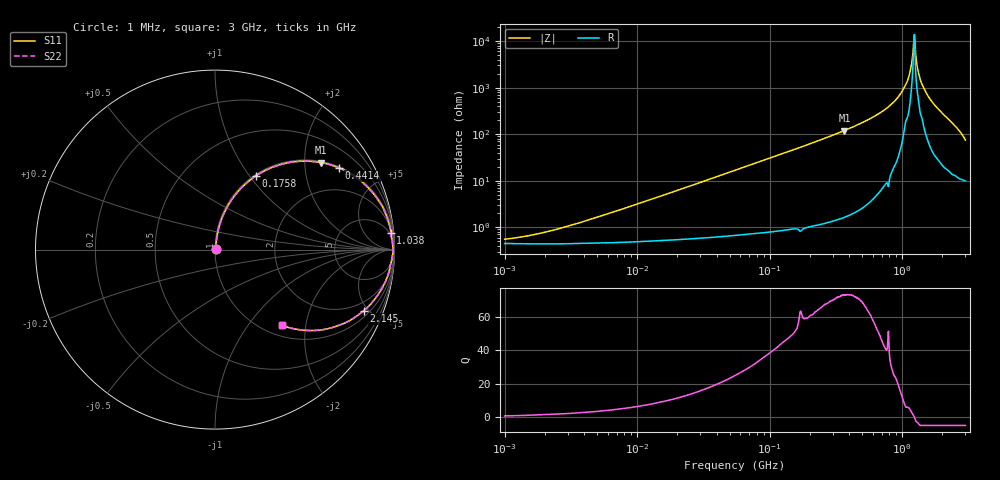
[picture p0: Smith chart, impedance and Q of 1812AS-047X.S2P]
!s-Parameter Generated by FASTRON Sdn. Bhd.
!FASTRON P/N : 1812AS-047X
!Keysight Technologies,E4991B,MY54100416,A.01.15
!Date created: Fri Oct 13 14:09:02 2023
!Version  : Rev00 Fri Oct 13 14:09:02 2023
!Data & Calibration Information:
!Freq	S11	S21	S12	S22
!PortZ  Port1:50+j0  Port2:50+j0
!When reading, reference impedance value at option line is always used.
! Remarks : This data is being provided solely for informational purposes.
# Hz S dB R 50
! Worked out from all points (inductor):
!   1601 points, 1 MHz to 3 GHz, reference 50 ohm
!   read as one part in series: L = 50.1 nH near 4.289 MHz
!   highest Q = 73.3 at 366.8 MHz (marker M1), where L = 52.1 nH
!   self-resonance near 1.231 GHz
!   S11 on the Smith chart (normalised r, x): 1 MHz: 1.01, +0.01; 175.8 MHz: 1.02, +1.08; 441.4 MHz: 1.04, +3.01; 1.038 GHz: 4, +20; 2.145 GHz: 1.36, -4.67; 3 GHz: 1.20, -1.48
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1000000  -45.18 35.6  -0.04 -0.2  -0.04 -0.2  -45.18 35.6
3804036  -37.85 68.9  -0.04 -0.7  -0.04 -0.7  -37.85 68.9
1.447069e7  -26.99 80.9  -0.05 -2.5  -0.05 -2.5  -26.99 80.9
5.477226e7  -15.73 78.3  -0.18 -9.4  -0.18 -9.4  -15.73 78.3
1.757585e8  -6.52 60.9  -1.17 -28.2  -1.17 -28.2  -6.52 60.9
2.083556e8  -5.39 56.5  -1.57 -32.5  -1.57 -32.5  -5.39 56.5
3.667557e8  -2.35 39.5  -3.93 -49.7  -3.93 -49.7  -2.35 39.5
4.413523e8  -1.64 33.4  -5.19 -55.8  -5.19 -55.8  -1.64 33.4
7.925923e8  -0.31 14.2  -12.23 -74.6  -12.23 -74.6  -0.31 14.2
9.209708e8  -0.18 9.3  -15.78 -77.9  -15.78 -77.9  -0.18 9.3
1.038491e9  -0.14 5.4  -20.40 -77.5  -20.40 -77.5  -0.14 5.4
1.125055e9  -0.10 3.2  -25.02 -76.4  -25.02 -76.4  -0.10 3.2
1.159346e9  -0.09 2.2  -28.23 -73.5  -28.23 -73.5  -0.09 2.2
1.200675e9  -0.08 1.0  -34.14 -62.0  -34.14 -62.0  -0.08 1.0
1.237271e9  -0.06 -0.1  -42.92 9.7  -42.92 9.7  -0.06 -0.1
1.268618e9  -0.07 -1.1  -33.72 66.2  -33.72 66.2  -0.07 -1.1
1.340405e9  -0.12 -2.9  -25.56 73.7  -25.56 73.7  -0.12 -2.9
1.45942e9  -0.17 -5.8  -19.84 75.8  -19.84 75.8  -0.17 -5.8
1.704314e9  -0.34 -11.7  -13.81 73.4  -13.81 73.4  -0.34 -11.7
2.145442e9  -0.96 -22.4  -8.35 63.2  -8.35 63.2  -0.96 -22.4
2.543347e9  -2.05 -33.1  -5.22 51.9  -5.22 51.9  -2.05 -33.1
3e9  -4.96 -48.4  -2.45 34.0  -2.45 34.0  -4.96 -48.4
